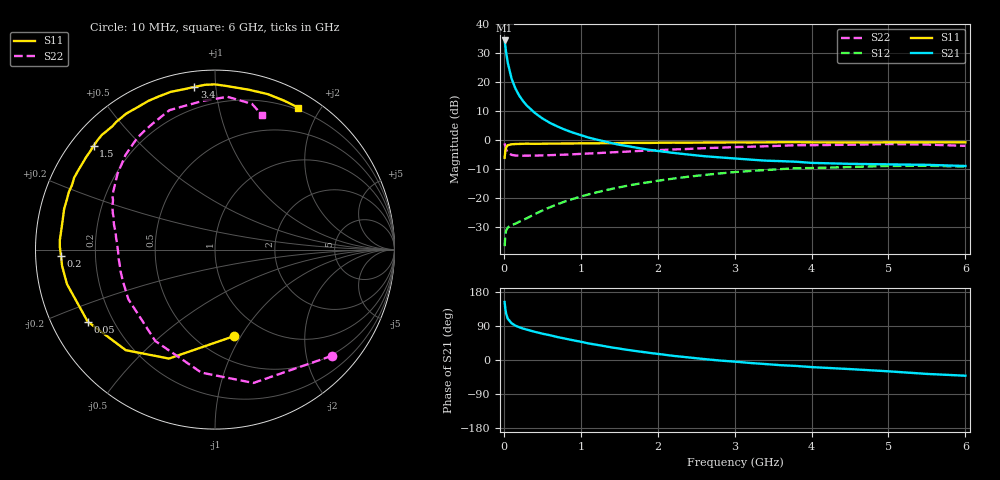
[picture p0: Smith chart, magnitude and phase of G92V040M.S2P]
! SIEMENS Small Signal Semiconductors
! BFG235
! Si NPN RF Bipolar Junction Transistor in SOT223
! VCE = 2 V  IC = 40 mA
! Common Emitter S-Parameters:  July  1994
# GHz  S  MA  R  50
!  f  S11  S21  S12  S22
! GHz  MAG  ANG  MAG  ANG  MAG  ANG  MAG  ANG
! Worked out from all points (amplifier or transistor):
!   40 points, 10 MHz to 6 GHz, reference 50 ohm
!   highest |S21| = 34.4 dB at 10 MHz (marker M1)
!   |S21| within 3 dB of that: start of sweep to 24.61 MHz
!   unconditionally stable (mu >= 1): 498.6 MHz to 1.5 GHz
!   at 200 MHz: K = 0.64, MSG = 21.8 dB, |S12| = -28.2 dB
!   at 1.5 GHz: K = 1.00, MAG = 7.3 dB, |S12| = -16.3 dB
!   at 6 GHz: K = 0.95, MSG = 0.1 dB, |S12| = -9.1 dB
!   S11 on the Smith chart (normalised r, x): 10 MHz: 0.73, -0.93; 50 MHz: 0.11, -0.26; 200 MHz: 0.08, -0.02; 1.5 GHz: 0.07, +0.37; 3.4 GHz: 0.08, +0.88; 6 GHz: 0.17, +1.73
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0.01  0.4938 -77.7  52.73 153.0  0.0147 64.2  0.8805 -42.2
0.02  0.6591 -112.9  41.58 134.3  0.023 48.2  0.7733 -73.9
0.03  0.7492 -131.6  32.91 122.3  0.0274 38.3  0.6896 -96.3
0.05  0.8148 -150.5  21.99 109.5  0.0309 29.1  0.6085 -123.1
0.1  0.8468 -166.9  11.66 97.0  0.034 26.6  0.5561 -150.3
0.15  0.8568 -173.9  7.827 90.7  0.0359 29.7  0.5423 -161.3
0.2  0.8586 -177.6  5.862 86.5  0.0389 33.6  0.5399 -167.3
0.25  0.8645 179.0  4.723 82.9  0.0417 37.1  0.5376 -171.4
0.3  0.8663 176.6  3.948 80.1  0.0447 40.1  0.5391 -174.5
0.4  0.863 171.8  2.97 74.5  0.0524 45.4  0.5399 -178.7
0.5  0.8655 168.0  2.374 69.5  0.0606 48.6  0.5442 178.1
0.6  0.8706 164.9  1.983 65.3  0.0691 50.7  0.5497 175.2
0.7  0.8711 161.4  1.712 60.4  0.0782 52.2  0.556 172.8
0.9  0.874 155.8  1.344 52.1  0.0964 52.4  0.5689 168.5
1.1  0.8806 149.3  1.107 43.8  0.1152 51.5  0.587 164.2
1.5  0.8897 139.5  0.831 30.1  0.1527 47.0  0.624 156.0
2.2  0.9048 123.1  0.602 11.0  0.2159 35.8  0.6893 141.8
3.2  0.91 101.4  0.461 -7.8  0.2925 16.4  0.7688 121.0
3.4  0.9136 97.2  0.442 -10.7  0.3036 12.2  0.7825 116.5
4.5  0.9104 78.0  0.389 -24.0  0.3426 -8.8  0.8317 94.5
5.5  0.9149 65.2  0.374 -36.7  0.3605 -26.8  0.8377 75.8
6  0.9171 59.6  0.357 -41.5  0.3491 -33.6  0.7955 70.9
